FUNCTION_BLOCK FB_AxisBase
VAR_INPUT

END_VAR
VAR_OUTPUT
	AlwayFalse			:	BOOL := FALSE;
	AlwayTrue			:	BOOL := TRUE;
END_VAR

VAR
	refAxis				: 	AXIS_REF;
	CamInStartMode		:	mc_startmode;
END_VAR

METHOD M_CamIn : BOOL
VAR_INPUT
	bExecute			:	BOOL;
	nMasterAxisId		:	UINT;
	nCamTableID			:	UDINT;
END_VAR
VAR_INST
	fbCamIn				:	MC_CamIn;
END_VAR
IF NOT AxisIsInVaild(nMasterAxisId) THEN 
	RETURN;
END_IF
fbCamIn(
	Master:= arAxis[nMasterAxisId].refAxis, 
	Slave:= refAxis, 
	Execute:= bExecute, 
	MasterOffset:= , 
	SlaveOffset:= , 
	MasterScaling:= , 
	SlaveScaling:= , 
	StartMode:= CamInStartMode, 
	CamTableID:= nCamTableID, 
	BufferMode:= , 
	Options:= , 
	InSync=> , 
	Busy=> , 
	Active=> , 
	CommandAborted=> , 
	Error=> , 
	ErrorID=> );
M_CamIn := fbCamIn.InSync;
END_METHOD

METHOD M_CamOut : BOOL
VAR_INPUT
	bExecute			:	BOOL;
END_VAR
VAR_INST
	fbCamOut			:	MC_CamOut;
END_VAR
fbCamOut(
	Slave:= refAxis, 
	Execute:= bExecute, 
	Options:= , 
	Done=> , 
	Busy=> , 
	Error=> , 
	ErrorID=> );
M_CamOut := fbCamOut.Done;
END_METHOD

METHOD M_GearIn : BOOL
VAR_INPUT
	bExecute			:	BOOL;
	fRatio				:	LREAL;
	nMasterAxisId		:	UINT;
END_VAR
VAR_INST
	fbGearIn			:	MC_GearIn;
END_VAR
IF NOT AxisIsInVaild(nMasterAxisId) THEN 
	RETURN;
END_IF

fbGearIn(
	Master:= arAxis[nMasterAxisId].refAxis, 
	Slave:= refAxis, 
	Execute:= bExecute, 
	RatioNumerator:= fRatio, 
	RatioDenominator:= 1, 
	Acceleration:= , 
	Deceleration:= , 
	Jerk:= , 
	BufferMode:= , 
	Options:= , 
	InGear=> , 
	Busy=> , 
	Active=> , 
	CommandAborted=> , 
	Error=> , 
	ErrorID=> );
	
M_GearIn := fbGearIn.InGear;
END_METHOD

METHOD M_GearOut : BOOL
VAR_INPUT
	bExecute			:	BOOL;
END_VAR
VAR_INST
	fbGearOut			:	MC_GearOut;
END_VAR
fbGearOut(
	Slave:= refAxis, 
	Execute:= bExecute, 
	Options:= , 
	Done=> , 
	Busy=> , 
	Error=> , 
	ErrorID=> );
	
M_GearOut := fbGearOut.Done;
END_METHOD

METHOD M_JogBackwards : BOOL
VAR_INPUT
	bExecute		:	BOOL;
END_VAR
VAR_INST
	fbJog				:	MC_Jog;
	
END_VAR
fbJog(
	Axis:= refAxis, 
	JogForward:= FALSE, 
	JogBackwards:= bExecute, 
	Mode:= , 
	Position:= , 
	Velocity:= , 
	Acceleration:= , 
	Deceleration:= , 
	Jerk:= , 
	Done=> , 
	Busy=> , 
	Active=> , 
	CommandAborted=> , 
	Error=> , 
	ErrorID=> );
END_METHOD

METHOD M_JogForward : BOOL
VAR_INPUT
	bExecute		:	BOOL;
	
END_VAR
VAR_INST
	fbJog				:	MC_Jog;
	
END_VAR
fbJog(
	Axis:= refAxis, 
	JogForward:= bExecute, 
	JogBackwards:= FALSE, 
	Mode:= , 
	Position:= , 
	Velocity:= , 
	Acceleration:= , 
	Deceleration:= , 
	Jerk:= , 
	Done=> , 
	Busy=> , 
	Active=> , 
	CommandAborted=> , 
	Error=> , 
	ErrorID=> );
END_METHOD

METHOD M_MovAbs : BOOL
VAR_INPUT
	bExecute			:	BOOL;
	fPosition			:	LREAL;
	fVelocity			:	LREAL;
END_VAR
VAR_INST
	fbMovAbs			:	MC_MoveAbsolute;
END_VAR
fbMovAbs(
	Axis:= refAxis, 
	Execute:= bExecute, 
	Position:= fPosition, 
	Velocity:= fVelocity, 
	Acceleration:= , 
	Deceleration:= , 
	Jerk:= , 
	BufferMode:= , 
	Options:= , 
	Done=> , 
	Busy=> , 
	Active=> , 
	CommandAborted=> , 
	Error=> , 
	ErrorID=> );
	
M_MovAbs := fbMovAbs.Done;
END_METHOD

METHOD M_MovRel : BOOL
VAR_INPUT
	bExecute			:	BOOL;
	fPosition			:	LREAL;
	fVelocity			:	LREAL;
END_VAR
VAR_INST
	fbMovRel		:	MC_MoveRelative;
END_VAR
fbMovRel(
	Axis:= refAxis, 
	Execute:= bExecute, 
	Distance:= fPosition, 
	Velocity:= fVelocity, 
	Acceleration:= , 
	Deceleration:= , 
	Jerk:= , 
	BufferMode:= , 
	Options:= , 
	Done=> , 
	Busy=> , 
	Active=> , 
	CommandAborted=> , 
	Error=> , 
	ErrorID=> );
M_MovRel := fbMovRel.Done;
END_METHOD

METHOD M_Power : BOOL
VAR_INPUT
	bExecute			:	BOOL;
	bEnable_Positive	:	BOOL;
	bEnable_Negative	:	BOOL;
	fOverride			:	LREAL;
END_VAR
VAR_INST
	fbPower				:	MC_Power;
END_VAR

fbPower(
	Axis:= refAxis, 
	Enable:= bExecute, 
	Enable_Positive:= bEnable_Positive, 
	Enable_Negative:= bEnable_Negative, 
	Override:= fOverride, 
	BufferMode:= , 
	Options:= , 
	Status=> , 
	Busy=> , 
	Active=> , 
	Error=> , 
	ErrorID=> );
M_Power := fbPower.Status;
END_METHOD

METHOD M_ReadStatus : BOOL
VAR_INPUT
END_VAR
refAxis.ReadStatus();
END_METHOD

METHOD M_Reset : BOOL
VAR_INPUT
	bExecute			:	BOOL;
END_VAR
VAR_INST
	fbNcReset			:	MC_Reset;
END_VAR
fbNcReset(
	Axis:= refAxis, 
	Execute:= bExecute, 
	Done=> , 
	Busy=> , 
	Error=> , 
	ErrorID=> );
M_Reset := fbNcReset.Done;
END_METHOD

METHOD M_SetPosition : BOOL
VAR_INPUT
	bExecute			:	BOOL;
	fPosition			:	LREAL;
END_VAR
VAR_INST
	fbSetPosition		:	MC_SetPosition;
END_VAR
fbSetPosition(
	Axis:= refAxis, 
	Execute:= bExecute, 
	Position:= fPosition, 
	Mode:= , 
	Options:= , 
	Done=> , 
	Busy=> , 
	Error=> , 
	ErrorID=> );
M_SetPosition := fbSetPosition.Done;
END_METHOD

METHOD M_Stop : BOOL
VAR_INPUT
	bExecute			:	BOOL;
END_VAR
VAR_INST
	fbStop				:	MC_Stop;
END_VAR
fbStop(
	Axis:= refAxis, 
	Execute:= bExecute, 
	Deceleration:= , 
	Jerk:= , 
	Options:= , 
	Done=> , 
	Busy=> , 
	Active=> , 
	CommandAborted=> , 
	Error=> , 
	ErrorID=> );
M_Stop := fbStop.Done;
END_METHOD

PROPERTY P_StartMode : mc_startmode
GET
P_StartMode := CamInStartMode;
END_GET
SET
CamInStartMode := P_StartMode;
END_SET
END_PROPERTY

END_FUNCTION_BLOCK
